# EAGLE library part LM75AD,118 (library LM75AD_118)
Board Mount Temperature Sensors I2C LOCAL +/- 2OC TS Source: Datasheet
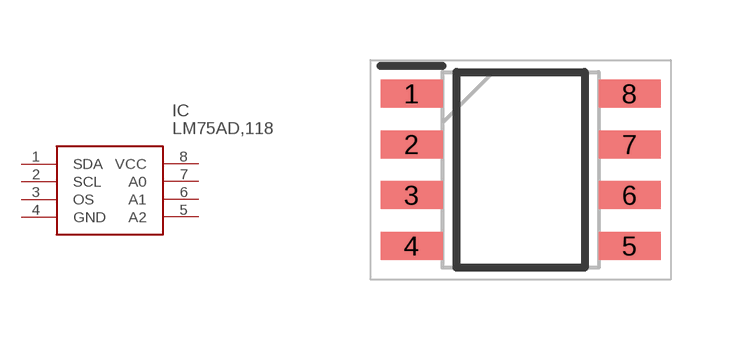
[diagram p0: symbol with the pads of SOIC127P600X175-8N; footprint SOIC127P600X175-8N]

Designator prefix IC

## LM75AD,118 (Arrow_Part_Number: LM75AD,118; Arrow_Price-Stock: https://www.arrow.com/en/products/lm75ad118/nxp-semiconductors?region=nac; Description: Board Mount Temperature Sensors I2C LOCAL +/- 2OC TS; Height: 1.75mm; Manufacturer_Name: NXP; Manufacturer_Part_Number: LM75AD,118; Mouser_Part_Number: 771-LM75AD-T; Mouser_Price-Stock: https://www.mouser.co.uk/ProductDetail/NXP-Semiconductors/LM75AD118?qs=LOCUfHb8d9tvtApDiOTqqg%3D%3D)  [SOIC127P600X175-8N]
1  SDA
2  SCL
3  OS
4  GND
5  A2
6  A1
7  A0
8  VCC

## Footprint SOIC127P600X175-8N (pad centres in mm)
SO8(1.75)
smd 1.55 x 0.7: 1 -2.725,1.905; 2 -2.725,0.635; 3 -2.725,-0.635; 4 -2.725,-1.905; 5 2.725,-1.905; 6 2.725,-0.635; 7 2.725,0.635; 8 2.725,1.905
